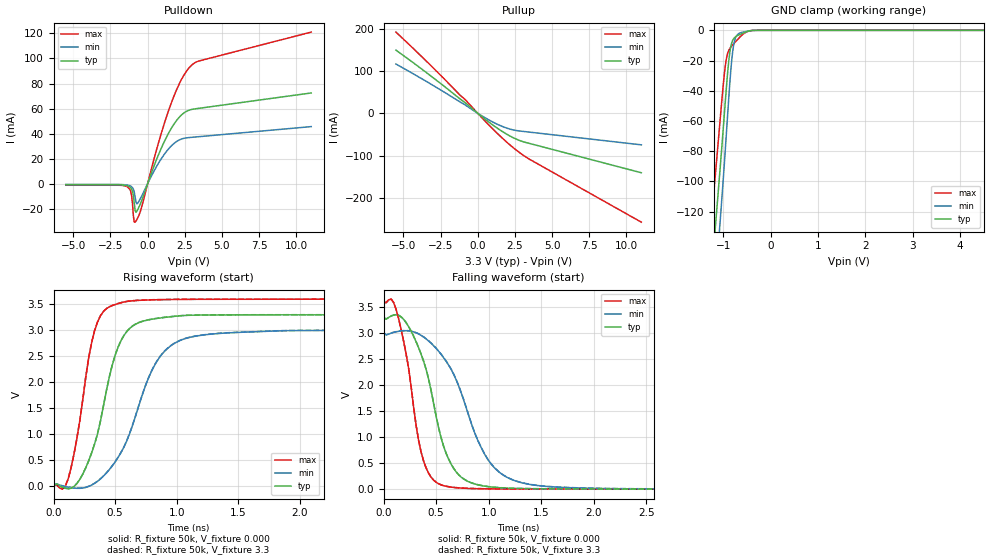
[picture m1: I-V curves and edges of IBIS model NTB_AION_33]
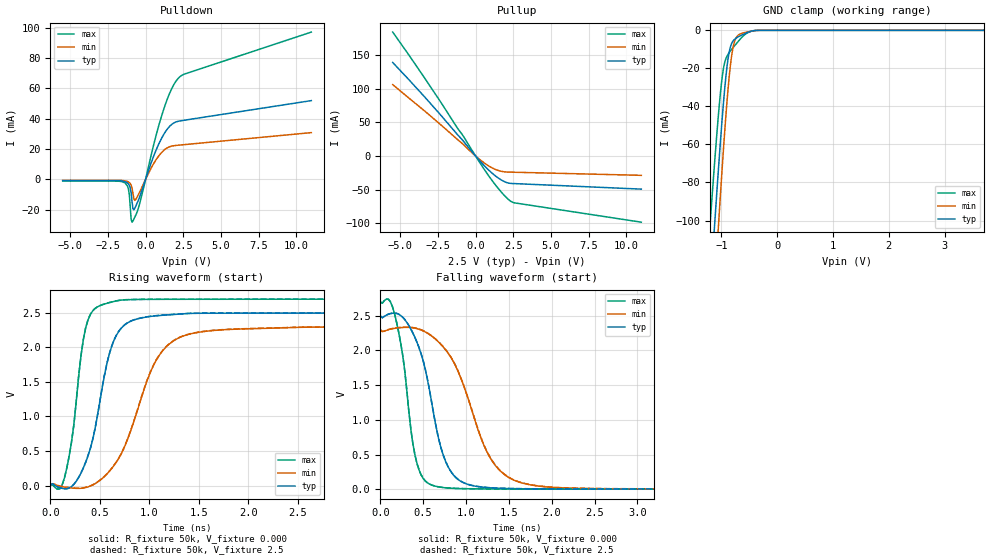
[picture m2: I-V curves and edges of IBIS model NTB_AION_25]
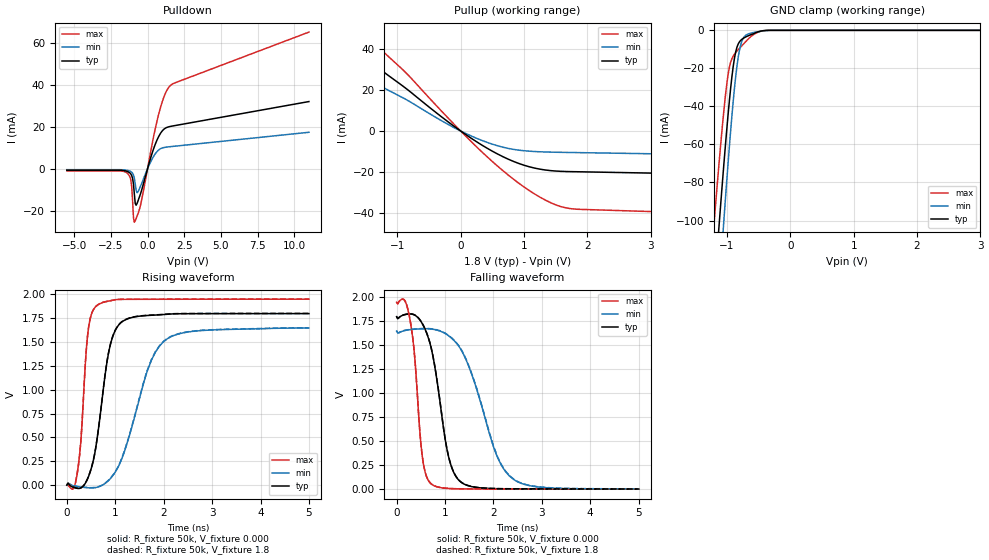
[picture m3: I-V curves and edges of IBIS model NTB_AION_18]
| NXP Semiconductors
| Logic Products Group
| IBIS model of NTB0104
| QUAD, DUAL-SUPPLY VOLTAGE-LEVEL TRANSLATING AUTO-DIRECTION SENSING
| TRANSCEIVER (3-STATE OE)
|[Packages]:
|[Package1]: DHVQFN14 (BQ) 14-pins package
|[Package2]: XQFN12 (GU12) 12-pins package
|[Package3]: WLSCP12 (UK) 12-bumps package
[IBIS Ver]   3.2
[File Name]   ntb0104.ibs
[File Rev]   1.1
[Date]   12-Dec-2011
[Source]   File created from simulations by LPG
   NXP Semiconductors Nijmegen
[Notes]   V1.1   Ibis model.
   Revision History
   Version Date   Author/Editor   Description
   1.0   May 2011   RRV   Initial Model
   1.1   December 2011  RRV   Added WLCSP12 package
   Remarks: - This type dynamically changes the output drive. Since the
   High-Drive determines the output edge, this model represents the
   output with High-Drive active only.
   - The Power Clamp curves have been omitted from the input
   since there is no power clamp diode.
   - IBISCHK 5.0.3 used
[Disclaimer]
   NXP Semiconductors warrants and represents that the IBIS model
   identified herein is owned by NXP Semiconductors (NXP). The
   model provided is not warranted as fully representing all of the
   operating characteristics and specifications of the semiconductor
   products to which the model relates.  Moreover, unless there is a
   signed, written agreement to the contrary, this IBIS model is
   furnished on an "as is" basis without support or warranty of any
   kind, either expressed or implied, regarding the use thereof, and
   NXP specifically disclaims all implied warranties of
   merchantability and fitness of the model for any purpose.
   NXP does not assume any liability arising out of the application
   or use of this IBIS model including infringement of patents and
   copyrights, nor does NXP convey any license under its patents and
   copyrights or the rights of others.
   NXP provides IBIS models as a service to our customers. You and
   your company shall not distribute, convey, sell, or give these models
   to anyone else without receiving prior written permission from
   NXP.
   NXP reserves the right to make changes without notice to these
   IBIS models to improve reliability, function, or design.
   Please be aware that your receipt and subsequent use of the IBIS
   information provided shall serve as acceptance of the terms and
   conditions of this agreement.  If you do not accept these terms,
   you should return or destroy the IBIS models and any other
   accompanying information immediately.
[Copyright]
   (C) Copyright 2011 NXP Semiconductors
   All rights reserved
|   Info for  DHVQFN14 (BQ) 14-pins package
[Component]   NTB0104_BQ
[Manufacturer]   NXP Semiconductors
[Package]
|   Typ   Min   Max
R_pkg   6.335E-02   5.611E-02   7.171E-02
L_pkg   9.743E-10   8.629E-10   1.103E-09
C_pkg   1.398E-13   1.323E-13   1.477E-13
[Pin] signal_name   model_name   R_pin   L_pin   C_pin
   1   VDDA   POWER 5.998E-02 9.226E-10 1.369E-13
   2   A1   NTB_AION 7.171E-02 1.103E-09 1.473E-13
   3   A2   NTB_AION 6.197E-02 9.530E-10 1.382E-13
   4   A3   NTB_AION 5.611E-02 8.629E-10 1.325E-13
   5   A4   NTB_AION 6.197E-02 9.529E-10 1.391E-13
   6   NC   NC 7.171E-02 1.103E-09 1.477E-13
   7   GND   GND 5.998E-02 9.227E-10 1.370E-13
   8   OE   NTB_CTRLIN 5.998E-02 9.226E-10 1.371E-13
   9   NC   NC 7.171E-02 1.103E-09 1.473E-13
   10   B4   NTB_BION 6.197E-02 9.531E-10 1.381E-13
   11   B3   NTB_BION 5.611E-02 8.630E-10 1.323E-13
   12   B2   NTB_BION 6.197E-02 9.530E-10 1.391E-13
   13   B1   NTB_BION 7.171E-02 1.103E-09 1.477E-13
   14   VDDB   POWER 5.998E-02 9.226E-10 1.370E-13
|   Info for  XQFN12 (GU12) 12-pins package
[Component]   NTB0104_GU12
[Manufacturer]   NXP Semiconductors
[Package]
|   Typ   Min   Max
R_pkg   4.874E-02   2.463E-02   6.249E-02
L_pkg   6.249E-10   3.157E-10   8.012E-10
C_pkg   5.624E-14   2.841E-14   7.211E-14
[Pin] signal_name   model_name   R_pin   L_pin   C_pin
   1   VDDA   POWER 6.001E-02 7.694E-10 6.924E-14
   2   A1   NTB_AION 4.620E-02 5.923E-10 5.331E-14
   3   A2   NTB_AION 4.197E-02 5.381E-10 4.843E-14
   4   A3   NTB_AION 4.855E-02 6.225E-10 5.602E-14
   5   A4   NTB_AION 6.249E-02 8.012E-10 7.211E-14
   6   GND   GND 2.463E-02 3.157E-10 2.841E-14
   7   B4   NTB_BION 6.117E-02 7.843E-10 7.059E-14
   8   B3   NTB_BION 4.602E-02 5.899E-10 5.309E-14
   9   B2   NTB_BION 3.808E-02 4.882E-10 4.394E-14
   10   B1   NTB_BION 4.179E-02 5.358E-10 4.822E-14
   11   VDDB   POWER 6.085E-02 7.802E-10 7.022E-14
   12   OEN   NTB_CTRLIN 5.312E-02 6.811E-10 6.130E-14
|   Info for  WLSCP12 (UK) 12-bumps package
[Component]   NTB0104_UK
[Manufacturer]   NXP Semiconductors
[Package]
|   Typ   Min   Max
R_pkg   3.558E-02   1.200E-02   1.610E-01
L_pkg   7.000E-11   5.000E-11   2.000E-10
C_pkg   7.000E-14   5.000E-14   2.000E-13
[Pin] signal_name   model_name   R_pin   L_pin   C_pin
   1   VDDA   POWER 1.300E-02 5.000E-11 5.000E-14
   2   A1   NTB_AION 1.200E-02 5.000E-11 5.000E-14
   3   A2   NTB_AION 1.200E-02 5.000E-11 5.000E-14
   4   A3   NTB_AION 1.300E-02 5.000E-11 5.000E-14
   5   A4   NTB_AION 8.600E-02 1.300E-10 1.300E-13
   6   GND   GND 2.600E-02 5.000E-11 5.000E-14
   7   B4   NTB_BION 2.400E-02 5.000E-11 5.000E-14
   8   B3   NTB_BION 2.400E-02 5.000E-11 5.000E-14
   9   B2   NTB_BION 2.500E-02 5.000E-11 5.000E-14
   10   B1   NTB_BION 1.700E-02 6.000E-11 6.000E-14
   11   VDDB   POWER 1.610E-01 2.000E-10 2.000E-13
   12   OEN   NTB_CTRLIN 1.400E-02 5.000E-11 5.000E-14
[Model Selector]   NTB_AION
NTB_AION_33   3.3V Vcc I/O model, non-inverting
NTB_AION_25   2.5V Vcc I/O model, non-inverting
NTB_AION_18   1.8V Vcc I/O model, non-inverting
[Model Selector]   NTB_BION
NTB_BION_50   5.0V Vcc I/O model, non-inverting
NTB_BION_33   3.3V Vcc I/O model, non-inverting
NTB_BION_25   2.5V Vcc I/O model, non-inverting
[Model Selector]   NTB_CTRLIN
NTB_CTRLIN_33   3.3V Vcc Input model
NTB_CTRLIN_25   2.5V Vcc Input model
NTB_CTRLIN_18   1.8V Vcc Input model
| Models and submodels in the file (9): NTB_AION_33 (I/O), NTB_AION_25 (I/O), NTB_AION_18 (I/O), NTB_CTRLIN_33 (Input), NTB_CTRLIN_25 (Input), NTB_CTRLIN_18 (Input), NTB_BION_50 (I/O), NTB_BION_33 (I/O), NTB_BION_25 (I/O)
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| Remark: If your software does not support the Model Selector
|   Please comment out the lines of the Model Selector, which
|   contain the name of the Model, except the one you want to use.
|   Model NTB_AION_33
[Model]   NTB_AION_33
Model_type   I/O
Polarity   Non-Inverting
Enable   Active-High
Vinh  =  2.145 | 0.65*Vcc
Vinl  =  1.116 | 0.35*Vcc
Vmeas =  1.65V | 0.5*Vcc
Cref  =  15e-12
Rref  =  50k
Vref  =  0V
C_comp   2.8130pF   2.5126pF   3.3706pF
[Model Spec]
| Note: The input and output voltage ratings may be exceeded if the input and
|   output current ratings are observed (please refer to the data sheet)
|   Subparameter   typ   min   max
Vinh   2.145   1.950   2.340
Vinl   1.116   1.050   1.260
| Overshoot
S_overshoot_high   6.5   6.5   6.5   | Static overshoot
S_overshoot_low   -0.5   -0.5   -0.5
D_overshoot_high   7.2   7.2   7.2   | Dynamic overshoot
D_overshoot_low   -1.0   -1.0   -1.0
D_overshoot_time   3n   3n   3n
| Timing Thresholds
Vmeas   1.65   1.5   1.8
|Ambient temperature:   25   85   -40
[Temperature Range]   40   100   -25
[Voltage Range]   3.3   3.0   3.6
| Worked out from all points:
|   slope of the pulldown table from 0 to 0.495 V, typ, clamps not added: 30.7 ohm
|   slope of the pullup table from 0 to 0.495 V, typ, clamps not added: 35.4 ohm
|   GND clamp passes 1 mA (typ) near -0.52 V on its own axis
|   rising waveform, R_fixture 50k, V_fixture 0.000: 20-80 % time 205ps typ, 301ps min, 147ps max; typ from 0 V to 3.3 V
|   rising waveform, R_fixture 50k, V_fixture 3.3: 20-80 % time 205ps typ, 300ps min, 147ps max; typ from 0.002 V to 3.3 V
|   falling waveform, R_fixture 50k, V_fixture 0.000: 20-80 % time 253ps typ, 369ps min, 170ps max; typ from 3.3 V to 0.001 V
|   falling waveform, R_fixture 50k, V_fixture 3.3: 20-80 % time 253ps typ, 369ps min, 170ps max; typ from 3.3 V to 0.003 V
|Process Range   nominal   slow   fast
[Pulldown]
|   voltage   I(typ)   I(min)   I(max)
-5.5V     -858.2uA   -592uA     -1.218mA
-1.36V    -1.662mA   -1.096mA   -2.469mA
-1.14V    -3.192mA   -1.899mA   -6.001mA
-1.02V    -5.874mA   -3.062mA   -15.31mA
-900mV    -15.24mA   -6.524mA   -30.64mA
-840mV    -21.45mA   -10.57mA   -30.72mA
-660mV    -20.58mA   -15.44mA   -27.21mA
574mV     18.51mA    13.16mA    25.99mA
1.476V    41.78mA    28.7mA     60.62mA
2.214V    54.16mA    35.4mA     81.77mA
2.87V     59.03mA    36.95mA    93.62mA
11V       72.47mA    45.6mA     121.1mA
[Pullup]
|   voltage   I(typ)   I(min)   I(max)
-5.5V     149mA      116.3mA    191.6mA
-3.35V    93.35mA    73.07mA    119.5mA
-1.2V     34.08mA    27mA       43.15mA
-840mV    24.87mA    19.55mA    32.02mA
666.7mV   -18.64mA   -14.08mA   -24.7mA
1.583V    -41.44mA   -30.06mA   -56.35mA
2.333V    -56.68mA   -38.81mA   -79.63mA
2.917V    -65.49mA   -42.23mA   -95.54mA
3.5V      -71.35mA   -44.55mA   -108.9mA
11V       -140.4mA   -74.49mA   -257mA
[GND_clamp]
|   voltage   I(typ)   I(min)   I(max)
-5.5V     -2.271A    -2.524A    -2.083A
-1.65V    -351.6mA   -411.8mA   -298.6mA
-1.2V     -143.1mA   -181.9mA   -107.7mA
-1.16V    -127.6mA   -165.2mA   -93.18mA
-1.08V    -96.85mA   -132.5mA   -64.36mA
-1.06V    -89.03mA   -124.2mA   -57.15mA
-960mV    -48.51mA   -80.51mA   -24.31mA
-860mV    -14.24mA   -34.4mA    -11.98mA
-780mV    -5.547mA   -9.614mA   -8.859mA
-640mV    -2.607mA   -1.683mA   -4.186mA
-340mV    -26.6uA    -37.53uA   -22.18uA
5.5V      0A         0A         0A
[Ramp]
| variable   typ   min   max
dV/dt_r  1.9777E+00/2.0527E-10  1.7971E+00/3.0050E-10  2.1584E+00/1.4687E-10
dV/dt_f  1.9778E+00/2.5275E-10  1.7971E+00/3.6860E-10  2.1586E+00/1.6960E-10
R_load = 50k
[Rising Waveform]
R_fixture   = 50k
V_fixture   = 0.000
V_fixture_min = 0.000
V_fixture_max = 0.000
| time   V(typ)   V(min)   V(max)
0s        1.169nV    11.72nV    36.72pV
119ps     -62.46mV   -31.59mV   129.9mV
190.5ps   41.74mV    -53.4mV    922.5mV
261.9ps   343.4mV    -35.83mV   2.099V
357.1ps   999.2mV    81.94mV    3.157V
523.8ps   2.671V     542.9mV    3.511V
642.9ps   3.081V     1.175V     3.566V
833.3ps   3.224V     2.377V     3.586V
1.119ns   3.287V     2.867V     3.593V
5ns       3.296V     2.995V     3.597V
[Rising Waveform]
R_fixture   = 50k
V_fixture   = 3.3
V_fixture_min = 3.0
V_fixture_max = 3.6
| time   V(typ)   V(min)   V(max)
0s        1.919mV    2.419mV    1.514mV
119ps     -60.51mV   -29.18mV   131.5mV
190.5ps   43.81mV    -50.94mV   924.4mV
261.9ps   345.8mV    -33.25mV   2.102V
357.1ps   1.002V     84.75mV    3.159V
523.8ps   2.675V     546.6mV    3.513V
642.9ps   3.084V     1.181V     3.568V
833.3ps   3.226V     2.383V     3.588V
1.119ns   3.29V      2.871V     3.595V
5ns       3.299V     2.998V     3.599V
[Falling Waveform]
R_fixture   = 50k
V_fixture   = 0.000
V_fixture_min = 0.000
V_fixture_max = 0.000
| time   V(typ)   V(min)   V(max)
0s        3.298V     2.997V     3.598V
119ps     3.35V      3.024V     3.45V
214.3ps   3.197V     3.044V     2.593V
285.7ps   2.936V     3.021V     1.57V
381ps     2.454V     2.922V     536.3mV
547.6ps   983.9mV    2.589V     82.04mV
714.3ps   276.5mV    1.984V     24.68mV
976.2ps   53.62mV    621.4mV    7.345mV
1.286ns   13.47mV    139.7mV    4.324mV
5ns       1.427mV    2.079mV    408uV
[Falling Waveform]
R_fixture   = 50k
V_fixture   = 3.3
V_fixture_min = 3.0
V_fixture_max = 3.6
| time   V(typ)   V(min)   V(max)
0s        3.3V       3V         3.6V
119ps     3.352V     3.026V     3.452V
214.3ps   3.2V       3.047V     2.596V
285.7ps   2.939V     3.024V     1.573V
381ps     2.457V     2.925V     538.6mV
547.6ps   988.4mV    2.593V     83.74mV
714.3ps   279.2mV    1.99V      26.25mV
976.2ps   55.73mV    626.9mV    8.872mV
1.286ns   15.45mV    142.8mV    5.841mV
5ns       3.348mV    4.5mV      1.923mV
|   Model NTB_AION_25
[Model]   NTB_AION_25
Model_type   I/O
Polarity   Non-Inverting
Enable   Active-High
Vinh  =  1.625 | 0.65*Vcc
Vinl  =  0.875 | 0.35*Vcc
Vmeas =  1.25V | 0.5*Vcc
Cref  =  15e-12
Rref  =  50k
Vref  =  0V
C_comp   2.8697pF   2.5695pF   3.4415pF
[Model Spec]
| Note: The input and output voltage ratings may be exceeded if the input and
|   output current ratings are observed (please refer to the data sheet)
|   Subparameter   typ   min   max
Vinh   1.625   1.495   1.755
Vinl   0.875   0.805   0.945
| Overshoot
S_overshoot_high   6.5   6.5   6.5   | Static overshoot
S_overshoot_low   -0.5   -0.5   -0.5
D_overshoot_high   7.2   7.2   7.2   | Dynamic overshoot
D_overshoot_low   -1.0   -1.0   -1.0
D_overshoot_time   3n   3n   3n
| Timing Thresholds
Vmeas   1.25   1.15   1.35
|Ambient temperature:   25   85   -40
[Temperature Range]   35   95   -35
[Voltage Range]   2.5   2.3   2.7
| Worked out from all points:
|   slope of the pulldown table from 0 to 0.375 V, typ, clamps not added: 34.1 ohm
|   slope of the pullup table from 0 to 0.375 V, typ, clamps not added: 39.5 ohm
|   GND clamp passes 1 mA (typ) near -0.53 V on its own axis
|   rising waveform, R_fixture 50k, V_fixture 0.000: 20-80 % time 220ps typ, 363ps min, 136ps max; typ from 0 V to 2.5 V
|   rising waveform, R_fixture 50k, V_fixture 2.5: 20-80 % time 220ps typ, 363ps min, 136ps max; typ from 0.002 V to 2.5 V
|   falling waveform, R_fixture 50k, V_fixture 0.000: 20-80 % time 269ps typ, 425ps min, 167ps max; typ from 2.5 V to 0.001 V
|   falling waveform, R_fixture 50k, V_fixture 2.5: 20-80 % time 269ps typ, 426ps min, 167ps max; typ from 2.5 V to 0.003 V
|Process Range   nominal   slow   fast
[Pulldown]
|   voltage   I(typ)   I(min)   I(max)
-5.5V     -800.9uA   -543uA     -1.151mA
-1.36V    -1.539mA   -985.1uA   -2.38mA
-1.14V    -2.974mA   -1.703mA   -6.197mA
-1.08V    -3.924mA   -2.113mA   -9.978mA
-960mV    -8.815mA   -3.83mA    -26.22mA
-900mV    -14.46mA   -5.783mA   -28.26mA
-840mV    -19.31mA   -9.144mA   -27.48mA
-660mV    -17.9mA    -13.37mA   -23.77mA
1.024V    26.36mA    17.29mA    40.56mA
1.6V      35.04mA    21.56mA    56.89mA
2.176V    38.36mA    22.56mA    66.78mA
11V       51.99mA    30.86mA    97.21mA
[Pullup]
|   voltage   I(typ)   I(min)   I(max)
-5.5V     138.9mA    106.1mA    184.1mA
-4.425V   113.4mA    86.06mA    150mA
-2.275V   59.83mA    45.72mA    78.82mA
-1.2V     31.78mA    24.51mA    41.29mA
-780mV    21.36mA    16.42mA    28.34mA
500mV     -12.52mA   -9.087mA   -17.34mA
1V        -23.55mA   -16.47mA   -33.48mA
1.5V      -32.59mA   -21.48mA   -48.09mA
1.917V    -38.07mA   -23.49mA   -58.74mA
2.25V     -40.47mA   -23.94mA   -65.92mA
2.667V    -41.07mA   -24.16mA   -69.92mA
11V       -49.2mA    -28.72mA   -98.33mA
[GND_clamp]
|   voltage   I(typ)   I(min)   I(max)
-2V       -519.3mA   -597.1mA   -450.4mA
-1.2V     -136.9mA   -174.4mA   -100.5mA
-1.12V    -101.3mA   -134.8mA   -68.62mA
-1.06V    -75.61mA   -105.9mA   -46.5mA
-1.04V    -67.35mA   -96.56mA   -39.75mA
-980mV    -44mA      -69.5mA    -23.14mA
-880mV    -14.62mA   -30.38mA   -12.54mA
-820mV    -7.105mA   -13.96mA   -10.09mA
-780mV    -5.212mA   -7.443mA   -8.653mA
-660mV    -2.825mA   -1.855mA   -4.478mA
-340mV    -22.09uA   -31.89uA   -13.77uA
5.5V      0A         0A         0A
[Ramp]
| variable   typ   min   max
dV/dt_r  1.4980E+00/2.1969E-10  1.3774E+00/3.6326E-10  1.6186E+00/1.3638E-10
dV/dt_f  1.4980E+00/2.6895E-10  1.3774E+00/4.2529E-10  1.6188E+00/1.6734E-10
R_load = 50k
[Rising Waveform]
R_fixture   = 50k
V_fixture   = 0.000
V_fixture_min = 0.000
V_fixture_max = 0.000
| time   V(typ)   V(min)   V(max)
0s        710.6pV    8.761nV    8.576pV
166.7ps   -47.62mV   -27.31mV   250.5mV
309.5ps   178.2mV    -40.16mV   1.872V
381ps     428.5mV    -20.18mV   2.398V
523.8ps   1.413V     100.6mV    2.616V
619.1ps   2.01V      244mV      2.656V
738.1ps   2.309V     521.6mV    2.687V
1.071ns   2.457V     1.816V     2.695V
1.357ns   2.487V     2.171V     2.696V
5ns       2.497V     2.296V     2.698V
[Rising Waveform]
R_fixture   = 50k
V_fixture   = 2.5
V_fixture_min = 2.3
V_fixture_max = 2.7
| time   V(typ)   V(min)   V(max)
0s        1.603mV    2.116mV    1.194mV
166.7ps   -45.95mV   -25.18mV   251.8mV
309.5ps   180.2mV    -37.89mV   1.874V
381ps     430.8mV    -17.79mV   2.4V
523.8ps   1.417V     103.3mV    2.618V
619.1ps   2.014V     247.2mV    2.657V
738.1ps   2.311V     526.3mV    2.688V
1.048ns   2.456V     1.759V     2.697V
1.357ns   2.489V     2.175V     2.698V
5ns       2.499V     2.298V     2.699V
[Falling Waveform]
R_fixture   = 50k
V_fixture   = 0.000
V_fixture_min = 0.000
V_fixture_max = 0.000
| time   V(typ)   V(min)   V(max)
0s        2.498V     2.298V     2.699V
166.7ps   2.538V     2.319V     2.526V
261.9ps   2.478V     2.332V     1.927V
404.8ps   2.185V     2.322V     491.4mV
595.2ps   1.281V     2.212V     62mV
714.3ps   569.3mV    2.078V     26.73mV
881ps     168.2mV    1.771V     10.72mV
1.262ns   21.87mV    496.9mV    4.004mV
1.571ns   7.636mV    124.1mV    3.126mV
5ns       1.425mV    1.933mV    481.9uV
[Falling Waveform]
R_fixture   = 50k
V_fixture   = 2.5
V_fixture_min = 2.3
V_fixture_max = 2.7
| time   V(typ)   V(min)   V(max)
0s        2.5V       2.3V       2.7V
166.7ps   2.54V      2.322V     2.528V
261.9ps   2.48V      2.334V     1.93V
404.8ps   2.188V     2.325V     493.8mV
595.2ps   1.285V     2.215V     63.31mV
714.3ps   573mV      2.082V     27.99mV
881ps     170.5mV    1.776V     11.94mV
1.262ns   23.62mV    502.7mV    5.203mV
1.571ns   9.292mV    127.3mV    4.322mV
5ns       3.029mV    4.053mV    1.676mV
|   Model NTB_AION_18
[Model]   NTB_AION_18
Model_type   I/O
Polarity   Non-Inverting
Enable   Active-High
Vinh  =  1.170 | 0.65*Vcc
Vinl  =  0.630 | 0.35*Vcc
Vmeas =  0.9   | 0.5*Vcc
Cref  =  15e-12
Rref  =  50k
Vref  =  0V
C_comp   2.9455pF   2.6456pF   3.5494pF
[Model Spec]
| Note: The input and output voltage ratings may be exceeded if the input and
|   output current ratings are observed (please refer to the data sheet)
|   Subparameter   typ   min   max
Vinh   1.170   1.073   1.268
Vinl   0.630   0.578   0.683
| Overshoot
S_overshoot_high   6.5   6.5   6.5   | Static overshoot
S_overshoot_low   -0.5   -0.5   -0.5
D_overshoot_high   7.2   7.2   7.2   | Dynamic overshoot
D_overshoot_low   -1.0   -1.0   -1.0
D_overshoot_time   3n   3n   3n
| Timing Thresholds
Vmeas   0.9   0.825   0.975
|Ambient temperature:   25   85   -40
[Temperature Range]   35   95   -35
[Voltage Range]   1.8   1.65   1.95
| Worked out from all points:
|   slope of the pulldown table from 0 to 0.27 V, typ, clamps not added: 41.9 ohm
|   slope of the pullup table from 0 to 0.27 V, typ, clamps not added: 48.1 ohm
|   GND clamp passes 1 mA (typ) near -0.53 V on its own axis
|   rising waveform, R_fixture 50k, V_fixture 0.000: 20-80 % time 297ps typ, 581ps min, 150ps max; typ from 0 V to 1.8 V
|   rising waveform, R_fixture 50k, V_fixture 1.8: 20-80 % time 297ps typ, 580ps min, 150ps max; typ from 0.001 V to 1.8 V
|   falling waveform, R_fixture 50k, V_fixture 0.000: 20-80 % time 335ps typ, 625ps min, 182ps max; typ from 1.8 V to 0.001 V
|   falling waveform, R_fixture 50k, V_fixture 1.8: 20-80 % time 335ps typ, 626ps min, 182ps max; typ from 1.8 V to 0.003 V
|Process Range   nominal   slow   fast
[Pulldown]
|   voltage   I(typ)   I(min)   I(max)
-5.5V     -719.9uA   -467.6uA   -1.062mA
-1.36V    -1.335mA   -806.4uA   -2.146mA
-1.14V    -2.519mA   -1.358mA   -5.416mA
-1.08V    -3.298mA   -1.673mA   -8.597mA
-960mV    -7.307mA   -3mA       -23.34mA
-900mV    -12.12mA   -4.527mA   -25.43mA
-840mV    -16.56mA   -7.232mA   -24.78mA
-660mV    -15.5mA    -11.05mA   -21.51mA
588mV     12.71mA    7.651mA    20.98mA
1.078V    18.53mA    10.01mA    33.4mA
1.519V    20.04mA    10.46mA    39.29mA
11V       31.93mA    17.32mA    64.96mA
[Pullup]
|   voltage   I(typ)   I(min)   I(max)
-5.5V     130.1mA    97.36mA    172mA
-3.35V    78.07mA    59.15mA    107mA
-2.275V   53.56mA    39.11mA    73.36mA
-1.2V     28.43mA    20.84mA    38.11mA
-840mV    20.21mA    14.98mA    27.67mA
-60mV     1.329mA    935.9uA    1.904mA
500mV     -9.85mA    -6.437mA   -14.86mA
833.3mV   -14.84mA   -8.993mA   -23.49mA
1.167V    -18.1mA    -10.03mA   -30.7mA
1.417V    -19.34mA   -10.33mA   -34.92mA
1.667V    -19.79mA   -10.47mA   -37.52mA
11V       -25.1mA    -15.04mA   -47.08mA
[GND_clamp]
|   voltage   I(typ)   I(min)   I(max)
-5.5V     -2.228A    -2.484A    -2.019A
-1.2V     -136.9mA   -174.4mA   -100.5mA
-1.12V    -101.3mA   -134.8mA   -68.62mA
-1.06V    -75.61mA   -105.9mA   -46.5mA
-1.04V    -67.35mA   -96.56mA   -39.75mA
-960mV    -36.89mA   -60.93mA   -19.41mA
-880mV    -14.62mA   -30.38mA   -12.54mA
-820mV    -7.105mA   -13.96mA   -10.09mA
-740mV    -4.18mA    -4.079mA   -7.271mA
-620mV    -2.282mA   -1.439mA   -3.26mA
-340mV    -22.09uA   -31.89uA   -13.77uA
5.5V      0A         0A         0A
[Ramp]
| variable   typ   min   max
dV/dt_r  1.0782E+00/2.9737E-10  9.8736E-01/5.8131E-10  1.1688E+00/1.4992E-10
dV/dt_f  1.0782E+00/3.3501E-10  9.8747E-01/6.2490E-10  1.1689E+00/1.8232E-10
R_load = 50k
[Rising Waveform]
R_fixture   = 50k
V_fixture   = 0.000
V_fixture_min = 0.000
V_fixture_max = 0.000
| time   V(typ)   V(min)   V(max)
0s        721.1pV    10.26nV    7.222pV
214.3ps   -33.72mV   -15.16mV   124.1mV
285.7ps   -30.33mV   -19.83mV   440.2mV
428.6ps   67.52mV    -27mV      1.571V
619.1ps   466mV      -22.74mV   1.88V
881ps     1.434V     59.67mV    1.929V
1.167ns   1.72V      321.7mV    1.946V
1.667ns   1.777V     1.204V     1.947V
2.083ns   1.79V      1.536V     1.947V
5ns       1.797V     1.646V     1.948V
[Rising Waveform]
R_fixture   = 50k
V_fixture   = 1.8
V_fixture_min = 1.65
V_fixture_max = 1.95
| time   V(typ)   V(min)   V(max)
0s        1.388mV    1.956mV    970.9uV
214.3ps   -32.25mV   -13.19mV   125.3mV
285.7ps   -28.77mV   -17.82mV   442mV
428.6ps   69.39mV    -24.85mV   1.573V
619.1ps   469.6mV    -20.34mV   1.881V
881ps     1.438V     62.72mV    1.931V
1.167ns   1.723V     327.1mV    1.947V
1.667ns   1.779V     1.211V     1.948V
2.083ns   1.792V     1.54V      1.948V
5ns       1.799V     1.648V     1.949V
[Falling Waveform]
R_fixture   = 50k
V_fixture   = 0.000
V_fixture_min = 0.000
V_fixture_max = 0.000
| time   V(typ)   V(min)   V(max)
0s        1.798V     1.648V     1.949V
261.9ps   1.827V     1.662V     1.808V
357.1ps   1.819V     1.667V     1.471V
523.8ps   1.732V     1.672V     370.7mV
714.3ps   1.473V     1.669V     56.04mV
1.071ns   343.9mV    1.601V     7.72mV
1.357ns   64.4mV     1.431V     3.583mV
2.083ns   5.49mV     333.4mV    2.12mV
2.417ns   3.235mV    102.2mV    1.854mV
5ns       1.404mV    2.058mV    651.6uV
[Falling Waveform]
R_fixture   = 50k
V_fixture   = 1.8
V_fixture_min = 1.65
V_fixture_max = 1.95
| time   V(typ)   V(min)   V(max)
0s        1.8V       1.65V      1.95V
261.9ps   1.829V     1.664V     1.81V
357.1ps   1.821V     1.669V     1.473V
523.8ps   1.734V     1.675V     372.8mV
714.3ps   1.476V     1.672V     57.23mV
1.071ns   348.1mV    1.604V     8.73mV
1.357ns   66.4mV     1.437V     4.567mV
2.083ns   6.928mV    340.8mV    3.092mV
2.417ns   4.656mV    106.2mV    2.826mV
5ns       2.794mV    4.043mV    1.623mV
